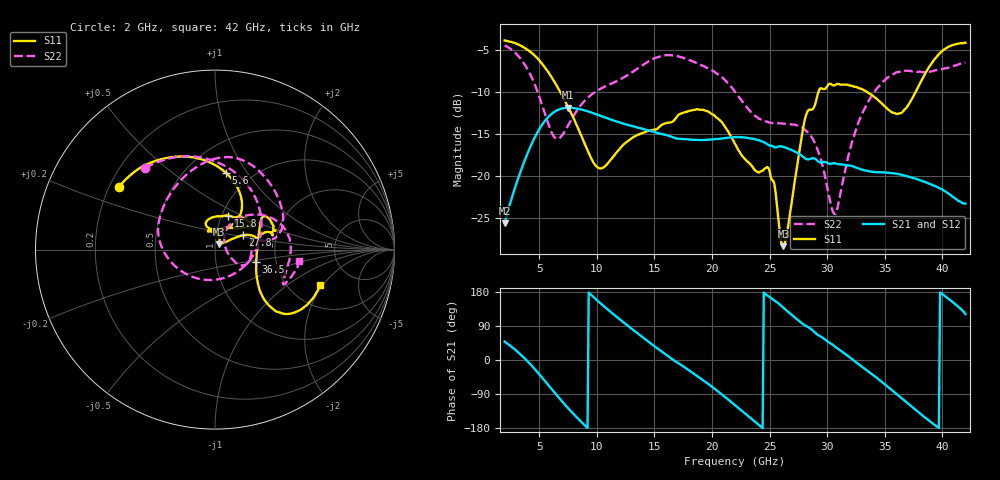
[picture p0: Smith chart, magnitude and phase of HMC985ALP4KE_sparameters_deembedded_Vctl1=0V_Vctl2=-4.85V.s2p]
!s2p File: Measurements: S11, S21, S12, S22
# GHz S dB R 50.0
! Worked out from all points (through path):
!   401 points, 2 GHz to 42 GHz, reference 50 ohm
!   highest |S21| = -11.90 dB at 7.5 GHz (marker M1); lowest = -25.7 dB at 2 GHz (marker M2)
!   lowest |S11| = -28.4 dB at 26.2 GHz (marker M3), VSWR 1.08, Z = 52.3 + j3.17 ohm
!   |S11| at or under -10 dB: 6.819 GHz to 29.25 GHz (22.43 GHz wide, 124 % of centre); 33.42 GHz to 37.69 GHz (4.269 GHz wide, 12 % of centre)
!   |S22| runs from -24.6 to -4.5 dB; largest |S21 - S12| = 0.00023
!   S11 on the Smith chart (normalised r, x): 2 GHz: 0.24, +0.28; 5.6 GHz: 0.76, +0.80; 15.8 GHz: 1.07, +0.42; 27.8 GHz: 1.34, +0.22; 36.5 GHz: 1.57, -0.23; 42 GHz: 2.94, -1.89
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2  -3.88 147.0  -25.67 48.6  -25.67 48.6  -4.47 130.5
3.6  -4.66 120.3  -18.70 8.4  -18.70 8.4  -6.47 84.9
4.7  -5.80 99.5  -15.22 -26.8  -15.22 -26.8  -9.40 43.4
5.6  -7.29 81.9  -13.30 -59.0  -13.30 -59.0  -13.03 -3.6
6.5  -9.22 66.5  -12.25 -91.9  -12.25 -91.9  -15.59 -68.7
7.5  -11.76 55.4  -11.90 -126.7  -11.90 -126.7  -14.03 -131.1
8.7  -15.38 55.1  -12.12 -164.6  -12.12 -164.6  -11.46 -170.1
10.4  -19.12 89.6  -12.90 147.6  -12.90 147.6  -9.58 162.5
15.4  -14.23 75.7  -14.97 27.6  -14.97 27.6  -5.81 87.3
15.8  -13.84 68.7  -15.07 18.7  -15.07 18.7  -5.67 82.3
19.4  -12.23 33.3  -15.73 -57.0  -15.73 -57.0  -7.03 35.3
22  -16.18 51.1  -15.40 -119.1  -15.41 -119.1  -9.99 9.8
24.9  -19.04 104.8  -16.33 168.2  -16.33 168.2  -13.61 13.2
26.2  -28.39 52.8  -16.56 137.8  -16.57 137.8  -13.80 -2.2
27.8  -15.23 27.2  -17.63 97.3  -17.63 97.3  -14.21 -24.1
28.7  -12.11 12.5  -17.92 79.2  -17.93 79.1  -15.48 -31.1
30.7  -9.21 20.7  -18.52 34.9  -18.52 34.9  -24.56 20.4
32.8  -9.59 33.9  -19.17 -12.7  -19.17 -12.7  -13.36 53.7
35.4  -12.21 11.8  -19.65 -73.9  -19.66 -73.9  -8.18 21.8
36.5  -12.48 -16.6  -19.90 -101.7  -19.91 -101.7  -7.52 7.7
39.5  -5.85 -43.8  -21.31 -175.0  -21.32 -175.0  -7.41 -26.4
42  -4.16 -18.6  -23.32 121.0  -23.33 121.0  -6.49 -7.5
